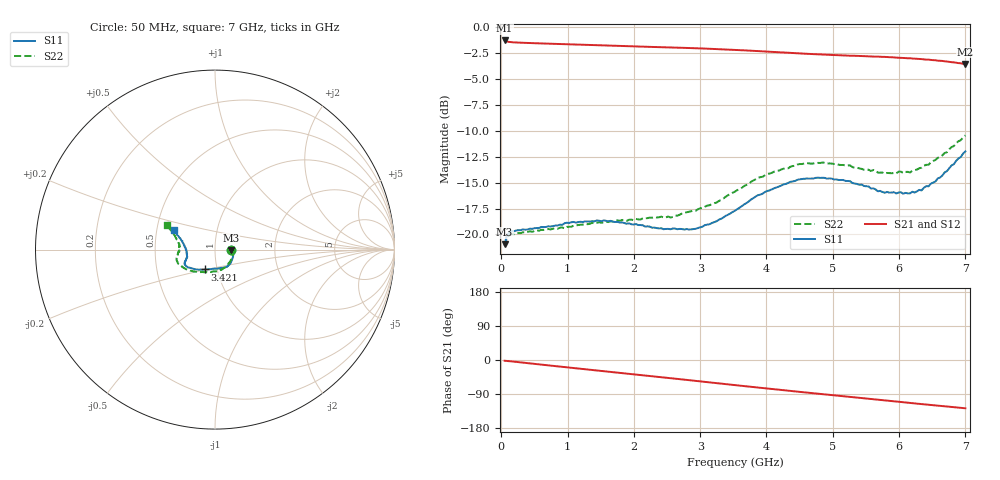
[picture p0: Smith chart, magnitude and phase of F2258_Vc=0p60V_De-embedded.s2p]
! Integrated Device Technology
! Corporate Headquarters
! 6024 Silver Creek Valley Road
! San Jose, CA 95138  USA
! Phone:  1-408-284-8200
! Toll Free:  1-800-223-1366
! Webpage:  http://www.idt.com/
! Timing and RF Division
! 515 Groton Road, Suite 102
! Westford, MA 01886-6024
! Device:  F2258
! Description: Voltage Variable RF Attenuator
! Frequency:  50.0 -  6000.00 MHz
! Package:  3x3 mm Thin QFN Plastic Package: 16 pin
! Ports:  2 RF, 2 DC
!  Pin  1  = NC
!  Pin  2  = NC
!  Pin  3  = RF2  = Port 2
!  Pin  4  = GND
!  Pin  5  = Vdd
!  Pin  6  = NC
!  Pin  7  = VCTRL
!  Pin  8  = NC
!  Pin  9  = GND
!  Pin 10  = RF1  = Port 1
!  Pin 11  = NC
!  Pin 12  = NC
!  Pin 13  = NC
!  Pin 14  = NC
!  Pin 15  = NC
!  Pin 16  = NC
! Vcntrl:  0.600 Volts
! Vdd:  +3.300 Volts
! Current:  1.108 mA
! Data:  The device was measured on a the F2258 evaluation board which has
!  individual transmission lines to the RF pins.  Data was collected
!  using a calibrated network analyzer.  The evaluation board was
!  de-embedded using a TRL calibration technique.
!  The reference plane is the edge of the package pin.
! Misc:  SN 10
!  Action Tracker AT0285
! Date Measured:  2014-12-10
! Date:  2016-01-13  MJV
! Note:
!  Integrated Device Technology supplies this data as a sample of measured
!  data at the package pin for this product.  Your particular data for this
!  product may vary.
!  Data was taken at 25 degrees C.
!  Integrated Device Technology reserves the right to change this data at anytime.
!Freq_(GHz)  S11M_(dB)  S11P_(deg)  S21M_(dB)  S21P_(deg)  S12M_(dB)  S12P_(deg)  S22M_(dB)  S22P_(deg)
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# GHz S dB R 50
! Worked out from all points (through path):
!   201 points, 50 MHz to 7 GHz, reference 50 ohm
!   highest |S21| = -1.27 dB at 50 MHz (marker M1); lowest = -3.6 dB at 7 GHz (marker M2)
!   group delay of S21, straight-line fit = 50.5 ps
!   lowest |S11| = -21.0 dB at 50 MHz (marker M3), VSWR 1.20, Z = 59.8 - j0.486 ohm
!   |S11| at or under -10 dB: start of sweep to end of sweep
!   |S22| runs from -21.1 to -10.4 dB; largest |S21 - S12| = 0.00077
!   S11 on the Smith chart (normalised r, x): 50 MHz: 1.20, -0.01; 3.421 GHz: 0.87, -0.20; 7 GHz: 0.62, +0.14
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0.05  -20.96 -2.6  -1.27 -2.0  -1.27 -2.0  -21.13 -2.8
0.08475  -20.10 -4.2  -1.37 -2.5  -1.38 -2.5  -20.30 -4.5
0.15425  -19.69 -6.6  -1.44 -3.7  -1.44 -3.7  -19.98 -7.9
0.71025  -19.21 -27.8  -1.58 -14.2  -1.58 -14.2  -19.47 -32.6
1.2315  -18.80 -46.0  -1.69 -23.9  -1.69 -23.9  -19.04 -55.1
1.6485  -18.68 -56.2  -1.78 -31.5  -1.78 -31.5  -18.73 -68.1
2.37825  -19.41 -73.5  -1.92 -44.8  -1.91 -44.8  -18.35 -87.2
2.552  -19.50 -78.9  -1.95 -48.0  -1.94 -48.0  -18.36 -92.5
2.93425  -19.45 -94.4  -2.03 -55.1  -2.02 -55.1  -17.70 -106.2
3.247  -18.72 -108.5  -2.10 -61.0  -2.10 -61.0  -16.92 -118.7
3.42075  -18.09 -117.2  -2.15 -64.3  -2.15 -64.3  -16.20 -125.8
3.525  -17.70 -121.2  -2.18 -66.3  -2.18 -66.2  -15.86 -129.7
4.0115  -15.80 -138.6  -2.36 -75.3  -2.36 -75.3  -14.16 -146.2
4.46325  -14.73 -148.6  -2.52 -83.5  -2.52 -83.5  -13.26 -158.0
4.7065  -14.59 -152.0  -2.59 -87.7  -2.60 -87.7  -13.15 -162.5
5.2625  -14.86 -158.3  -2.75 -97.4  -2.75 -97.4  -13.34 -171.1
5.6795  -15.83 -163.8  -2.84 -104.6  -2.84 -104.6  -14.03 -177.0
5.85325  -15.96 -168.0  -2.89 -107.7  -2.90 -107.7  -14.07 178.3
6.166  -16.03 -176.2  -2.99 -113.3  -3.00 -113.3  -14.02 172.0
6.33975  -15.74 176.6  -3.07 -116.4  -3.08 -116.4  -13.55 167.4
6.6525  -14.31 165.0  -3.25 -121.9  -3.26 -121.9  -12.36 160.4
7  -11.98 154.9  -3.55 -127.4  -3.56 -127.4  -10.44 152.8
